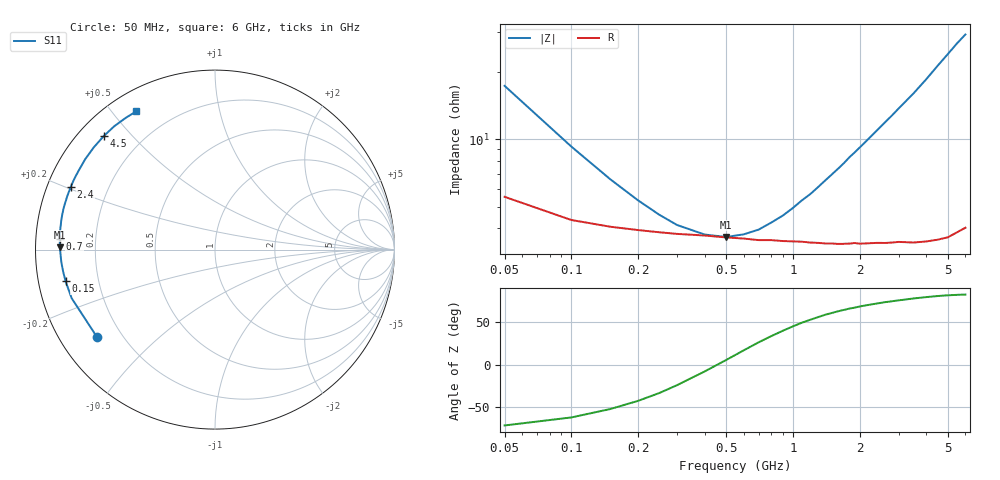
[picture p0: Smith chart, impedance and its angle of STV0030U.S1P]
! SIEMENS Discrete & RF Semiconductors
! BA892
! Si PIN Diode in SCD-80
! IF = 0.03 mA
! S-Parameters:  September  1997
# GHz  S  MA  R  50
!  f  S11
! GHz  MAG  ANG
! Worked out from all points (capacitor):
!   34 points, 50 MHz to 6 GHz, reference 50 ohm
!   read as one part to ground: C = 186 pF near 50 MHz
!   lowest |Z| = 3.66 ohm at 500 MHz (marker M1)
!   series resonance near 460 MHz, so ESL is about 650 pH
!   S11 on the Smith chart (normalised r, x): 50 MHz: 0.11, -0.33; 150 MHz: 0.08, -0.10; 700 MHz: 0.07, +0.03; 2.4 GHz: 0.07, +0.21; 4.5 GHz: 0.07, +0.42; 6 GHz: 0.08, +0.58
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0.05  0.8184 -143.4
0.1  0.8434 -161.3
0.15  0.8509 -168.0
0.2  0.8548 -171.7
0.25  0.8575 -174.2
0.3  0.8595 -176.1
0.4  0.8615 -178.8
0.5  0.864 179.2
0.6  0.8655 177.5
0.7  0.8676 176.0
0.8  0.8678 174.6
1.1  0.8703 170.7
1.2  0.8715 169.6
1.4  0.8731 167.2
1.6  0.8742 165.0
1.8  0.8745 162.7
1.9  0.8741 161.7
2  0.8753 160.6
2.4  0.8759 156.4
2.6  0.877 154.3
2.8  0.8775 152.3
3  0.8778 150.2
3.5  0.8813 145.2
4  0.8836 139.9
4.5  0.8857 134.4
5  0.8874 129.2
5.5  0.8867 124.1
6  0.8863 119.6
